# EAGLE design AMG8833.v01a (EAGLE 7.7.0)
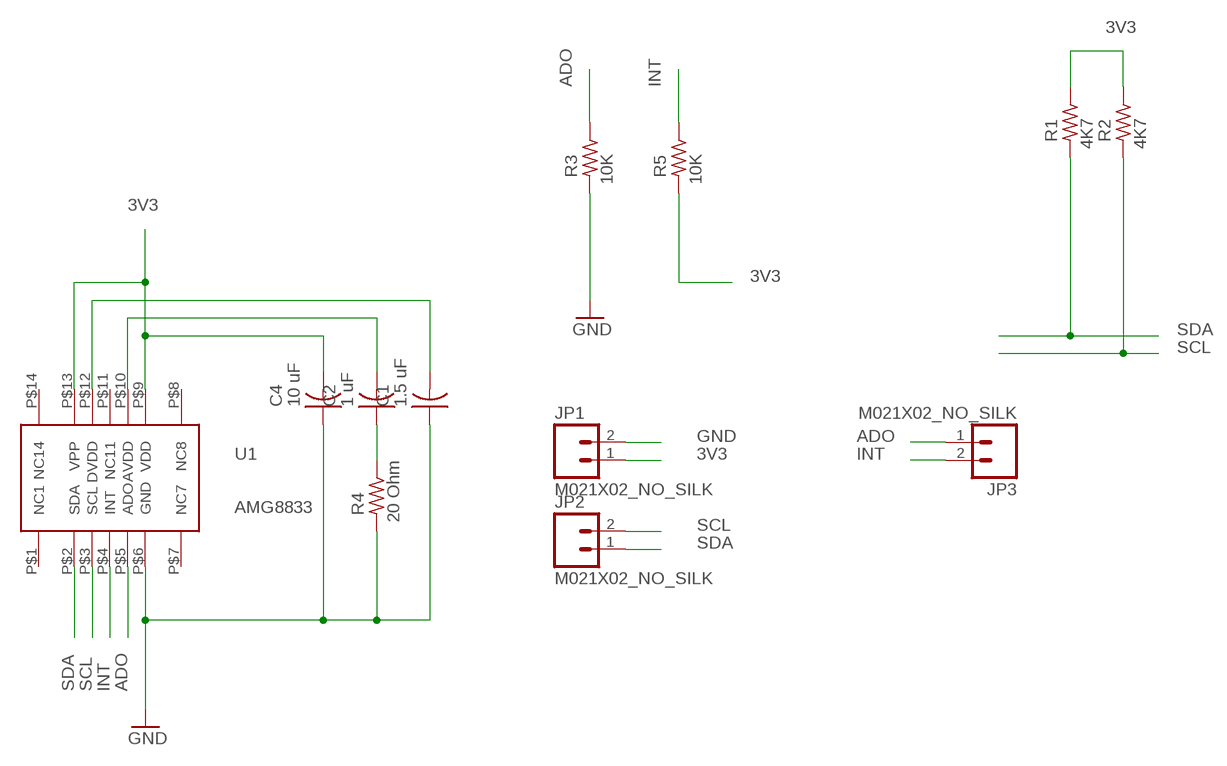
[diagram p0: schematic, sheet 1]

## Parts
C1  1.5 uF  C-US  [C0402_B]
C2  1 uF  C-US  [C0402_B]
C4  10 uF  C-US  [C0402_B]
JP1  M021X02_NO_SILK  [1X02_NO_SILK]
JP2  M021X02_NO_SILK  [1X02_NO_SILK]
JP3  M021X02_NO_SILK  [1X02_NO_SILK]
R1  4K7  R-US_  [R0402_B]
R2  4K7  R-US_  [R0402_B]
R3  10K  R-US_  [R0402_B]
R4  20 Ohm  R-US_  [R0402_B]
R5  10K  R-US_  [R0402_B]
U1  AMG8833  [AMG8833]

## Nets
3V3: C4.2 JP1.1 R1.1 R2.1 R5.2 U1.P$9(VDD) U1.P$13(VPP)
ADO: JP3.1 R3.1 U1.P$5(ADO)
GND: C1.1 C4.1 JP1.2 R3.2 R4.2 U1.P$6(GND)
INT: JP3.2 R5.1 U1.P$4(INT)
N$3: C1.2 U1.P$12(DVDD)
N$5: C2.2 U1.P$10(AVDD)
N$6: C2.1 R4.1
SCL: JP2.2 R2.2 U1.P$3(SCL)
SDA: JP2.1 R1.2 U1.P$2(SDA)
Unconnected: U1.P$1(NC1) U1.P$7(NC7) U1.P$8(NC8) U1.P$11(NC11) U1.P$14(NC14)

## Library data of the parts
C1 C2 C4 = Spark:C-US: Capacitor
JP1-JP3 = SparkFun-Connectors:M02: Standard 2-pin 0.1" header. Use with
R1-R5 = Spark:R-US_: 0402 Resistor
U1 = kris:AMG8833: Panasonic AMG8833 Grideye 8 x 8 IR Array https://na.industrial.panasonic.com/products/sensors/sensors-automotive-industrial-applications/grid-eye-infrared-array-sensor/series/grid-eye-high-performance-type-amg8833/ADI8005?reset=1

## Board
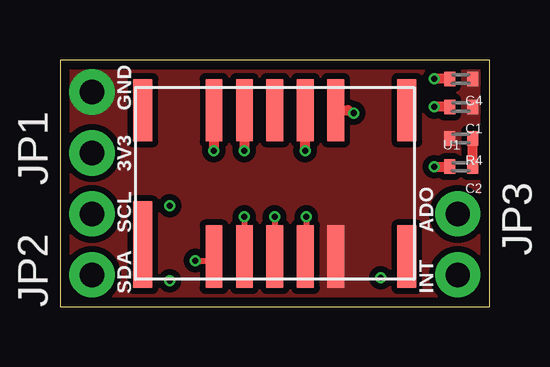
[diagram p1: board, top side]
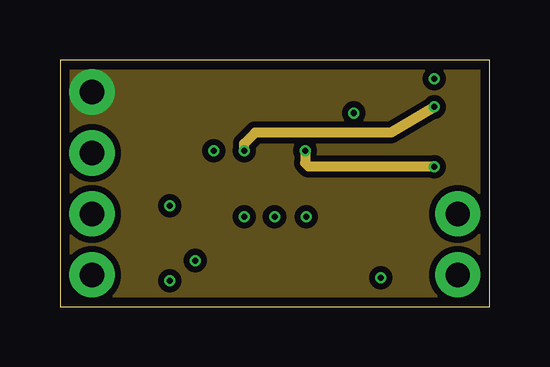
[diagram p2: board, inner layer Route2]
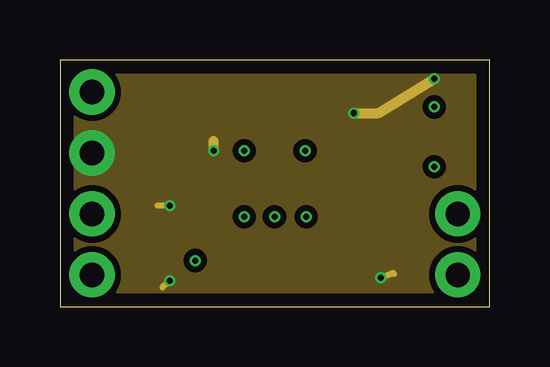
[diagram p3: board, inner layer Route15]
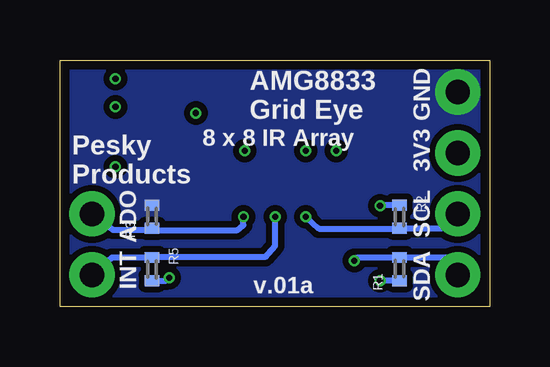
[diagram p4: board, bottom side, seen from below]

Size 17.91 x 10.29 mm. Coordinates in mm from the lower left corner, seen from the top.
Outline: 0,0 17.91,0 17.91,10.29 0,10.29 0,0
Copper layers (1*2*15*16): Top 0.035559375mm / dielectric 0.17018125mm / Route2 0.01778125mm / dielectric 47mil / Route15 0.01778125mm / dielectric 0.17018125mm / Bottom 0.035559375mm
Design rules "OSHPark-4layer *": minimum track width 5mil, minimum drill 10mil, track to track 5mil, track to pad 5mil, pad to pad 5mil, via to via 5mil, smd to smd 5mil, copper to edge 15mil, drill to drill 6mil, minimum pad ring 4mil, minimum via ring 4mil, stop-mask expansion 2.5mil, vias tented up to drill 20mil, thermal gap 10mil

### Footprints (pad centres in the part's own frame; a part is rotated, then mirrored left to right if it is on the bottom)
C0402_B = smd 0.457 x 0.61: 1 -0.483,0; 2 0.483,0
1X02_NO_SILK = drill 1.016 pad 1.88: 1 0,0; 2 2.54,0
R0402_B = smd 0.457 x 0.61: 1 -0.483,0; 2 0.483,0
AMG8833 = smd 0.8 x 3.6: P$1 -5.5,-2.55 | smd 0.7 x 2.6: P$2 -2.54,-3.05; P$3 -1.27,-3.05; P$4 0,-3.05; P$5 1.27,-3.05; P$6 2.54,-3.05; P$9 2.54,3.05; P$10 1.27,3.05; P$11 0,3.05; P$12 -1.27,3.05; P$13 -2.54,3.05 | smd 0.8 x 2.6: P$7 5.5,-3.05; P$8 5.5,3.05; P$14 -5.5,3.05

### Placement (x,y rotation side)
C1  16.71,8.33 180 top
C2  16.71,5.84 180 top
C4  16.71,9.5 180 top
JP1  1.33,6.41 90 top
JP2  1.33,1.33 90 top
JP3  16.57,3.87 270 top
R1  3.76,1.57 90 bottom
R2  3.76,3.76 270 bottom
R3  14.07,3.76 90 bottom
R4  16.71,7.01 180 top
R5  14.07,1.57 270 bottom
U1  8.95,5.14 0 top

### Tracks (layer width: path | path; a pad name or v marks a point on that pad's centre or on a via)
3V3  (via drill 0.25)
  Top 0.406: U1.P$13 6.41,6.51 v6.4,6.5 | U1.P$9 12,8.19 v12.24,8.08 | C4.2 v15.6,9.5
  Route15 0.254: v4.57,1.09 4.27,0.81 | v4.57,4.22 4.06,4.22 | v13.36,1.22 13.87,1.42 13.92,1.37
  Route15 0.406: v6.4,6.5 6.4,6.91 | v12.24,8.08 13.26,8.08 v15.6,9.5
  Bottom 0.254: R1.1 v4.57,1.09 | R2.1 4.5,4.24 v4.57,4.22 | R5.2 13.49,1.09 v13.36,1.22
  pour Route15 (isolate 0.254, no thermals): 0.64,9.65 17.27,9.65 17.27,0.64 0.64,0.64
ADO  (via drill 0.25)
  Top 0.254: v10.26,3.76 10.26,2 U1.P$5
  Bottom 0.254: JP3.1 15.71,3.21 14.14,3.21 R3.1 13.99,3.2 10.52,3.2 10.26,3.4 v10.26,3.76
GND
  pour Bottom (isolate 0.254, no thermals): 0,10.41 18.03,10.41 18.03,0 0,0
  pour Route2 (isolate 0.254, no thermals): 0,10.41 18.03,10.41 18.03,0 0,0
  pour Top (isolate 0.254, no thermals): 0,10.41 18.03,10.41 18.03,0 0,0
INT  (via drill 0.25)
  Top 0.254: v8.94,3.76 8.94,2.11 U1.P$4
  Bottom 0.254: v8.94,3.76 8.94,2.54 9.36,2.07 13.95,2.07 R5.1 15.75,2.06 JP3.2
N$3  (via drill 0.25)
  Top 0.406: U1.P$12 7.68,6.54 v7.67,6.5 | C1.2 v15.6,8.33
  Route2 0.406: v15.6,8.33 13.77,7.26 8.13,7.26 7.67,6.81 v7.67,6.5
N$5  (via drill 0.25)
  Top 0.254: 10.21,8.05 U1.P$10
  Top 0.406: v10.21,6.5 10.21,8.05 | v15.6,5.84 C2.2
  Route2 0.406: v15.6,5.84 10.36,5.84 10.21,5.99 v10.21,6.5
N$6
  Top 0.406: C2.1 R4.1
SCL  (via drill 0.25)
  Top 0.254: v7.67,3.76 7.67,2.11 U1.P$3
  Bottom 0.254: JP2.2 1.98,3.28 R2.2 3.79,3.26 7.12,3.26 v7.67,3.76
SDA  (via drill 0.25)
  Top 0.254: v5.64,1.93 6.25,1.93 U1.P$2
  Bottom 0.254: JP2.1 1.82,2.06 R1.2 5.51,2.06 v5.64,1.93

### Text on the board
tPlace: GND | 3V3 | SCL | ADO | SDA | INT
bPlace: GND | AMG8833 / Grid Eye | 3V3 | 8 x 8 IR Array | SCL | ADO | Pesky / Products | SDA | INT | v.01a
